PROGRAM Pro1

VAR
	{attribute 'OPC.UA.DA' := '1'}
	V1: INT;
	{attribute 'OPC.UA.DA' := '1'}
	B1: BOOL;
	{attribute 'OPC.UA.DA' := '1'}
	B2: BOOL;
	
	B3: BOOL;	// NO OPC UA Varible
	
	{attribute 'OPC.UA.DA' := '1'}
	W1:UINT;	
	{attribute 'OPC.UA.DA' := '1'}
	W2:WORD;
	W3:UINT;	// NO OPC UA Varible
	
	{attribute 'OPC.UA.DA' := '1'}
	D1,D2,D3:DWORD;	// Only the D1 is the OPC Varible
	
	{attribute 'OPC.UA.DA' := '1'}
	F1,F2,F3:REAL;	// Only the F1 is the OPC Varible
	F4:REAL;	// NO OPC UA Varible
	
	{attribute 'OPC.UA.DA' := '1'}
	S1,S2,S3:STRING;	// Only the S1 is the OPC Varible
	
	{attribute 'OPC.UA.DA' := '1'}
	WS1,WS2,WS3:WSTRING;	// Only the WS1 is the OPC Varible
	WS4:WSTRING;	// NO OPC UA Varible
	
	{attribute 'OPC.UA.DA' := '1'}
	ST1,ST2,ST3:CS1;	// Only the ST1 is the OPC Varible
	
	{attribute 'OPC.UA.DA' := '1'}
	arr1: ARRAY[1..9] OF LREAL;
	
	{attribute 'OPC.UA.DA' := '1'}
	B10: BOOL;
	
	{attribute 'OPC.UA.DA' := '1'}
	B11: BOOL;
	
	{attribute 'OPC.UA.DA' := '1'}
	Q1 AT %Q*: BOOL;
END_VAR

V1:=V1+1;
IF B1 THEN
	V1:=0;
	B1:=0;
END_IF

arr1[1]:=INT_TO_LREAL(v1);


IF B10 THEN
	Q1:=1;
	B10:=0;
END_IF
IF B11 THEN
	Q1:=0;
	B11:=0;
END_IF

END_PROGRAM
